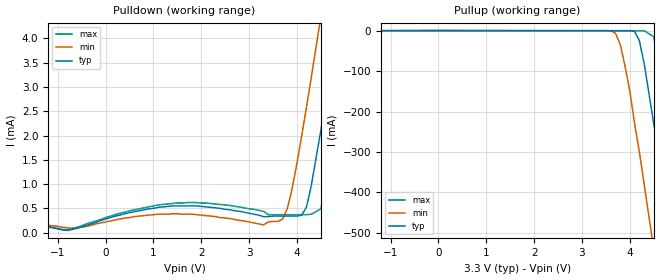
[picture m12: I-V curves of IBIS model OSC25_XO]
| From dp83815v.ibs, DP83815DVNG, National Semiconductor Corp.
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|   Model OSC25_XO
[Model]   OSC25_XO
Model_type   Output
Polarity   Inverting
Enable   Active-High
Vmeas =   1.50V
Cref =  10.00pF
Rref = 100.00k
C_comp   5.00pF   5.00pF   5.00pF
[Temperature Range]   25.00   0.14k   0.000
[Voltage Range]   3.30V   3.00V   3.60V
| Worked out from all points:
|   slope of the pulldown table from 0 to 0.495 V, typ, clamps not added: 3.84 kohm
|   slope of the pullup table from 0 to 0.495 V, typ, clamps not added: 5.7 kohm
[Pulldown]
| voltage   I(typ)   I(min)   I(max)
-3.3V     250uA      210uA      270uA
-800mV    46.06uA    100uA      59.79uA
1.7V      550uA      380uA      620uA
3.6V      340uA      230uA      370uA
3.9V      340uA      910uA      370uA
4.1V      360uA      2mA        370uA
4.3V      970uA      3.2mA      380uA
4.5V      2.11mA     4.45mA     490uA
4.9V      4.63mA     7.03mA     2.62mA
5.1V      5.93mA     8.34mA     3.89mA
5.3V      7.26mA     9.66mA     5.18mA
6.6V      16.11mA    18.46mA    13.95mA
[Pullup]
| voltage   I(typ)   I(min)   I(max)
-3.3V     -460uA     -400uA     -500uA
3.6V      -280uA     -810uA     -310uA
3.8V      -290uA     -34.42mA   -310uA
3.9V      -290uA     -87.92mA   -310uA
4.1V      -2.2mA     -230mA     -320uA
4.3V      -81.65mA   -380mA     -330uA
4.5V      -230mA     -540mA     -15.13mA
4.7V      -380mA     -700mA     -140mA
4.9V      -540mA     -860mA     -290mA
5.1V      -710mA     -1.02A     -450mA
5.3V      -870mA     -1.19A     -610mA
6.6V      -1.96A     -2.27A     -1.69A
[Ramp]
| variable   typ   min   max
dV/dt_r   1.17/12.24n   0.95/14.20n   1.30/11.52n
dV/dt_f   1.35/9.04n   1.02/12.21n   1.49/8.41n
R_load = 10.00k
| End [Model] OSC25_XO
